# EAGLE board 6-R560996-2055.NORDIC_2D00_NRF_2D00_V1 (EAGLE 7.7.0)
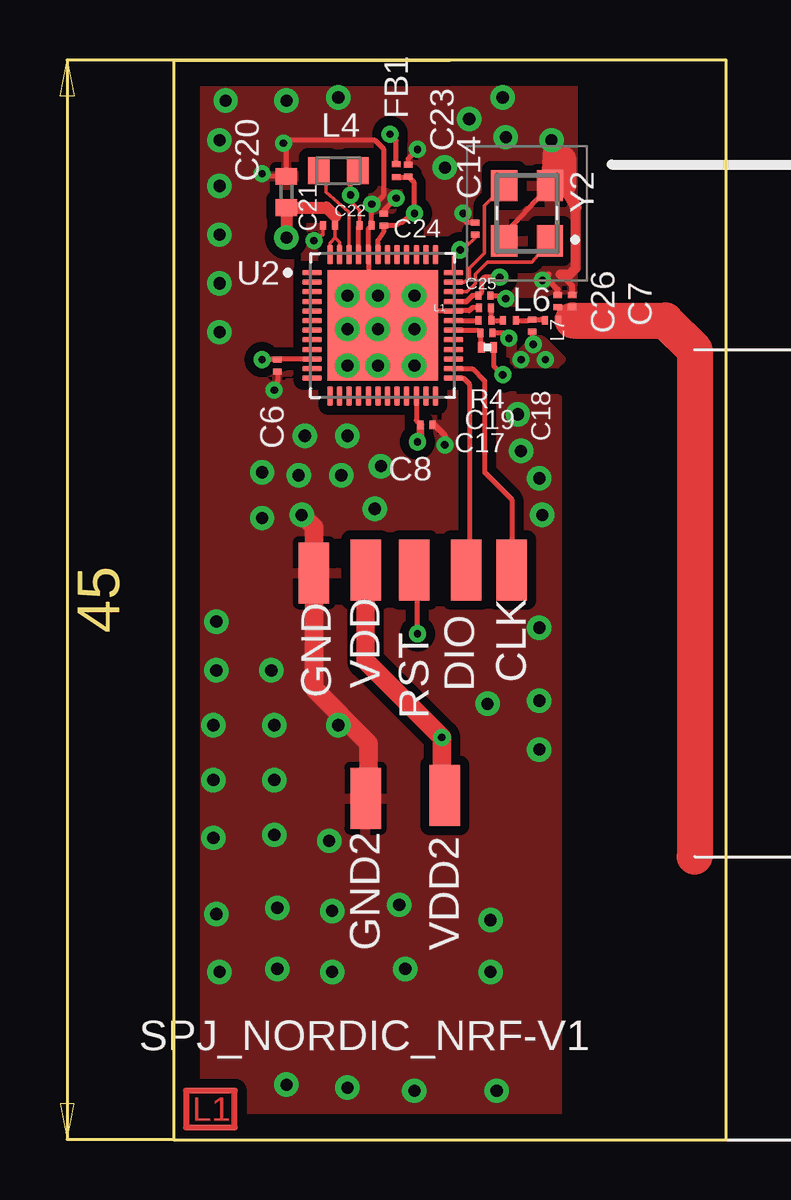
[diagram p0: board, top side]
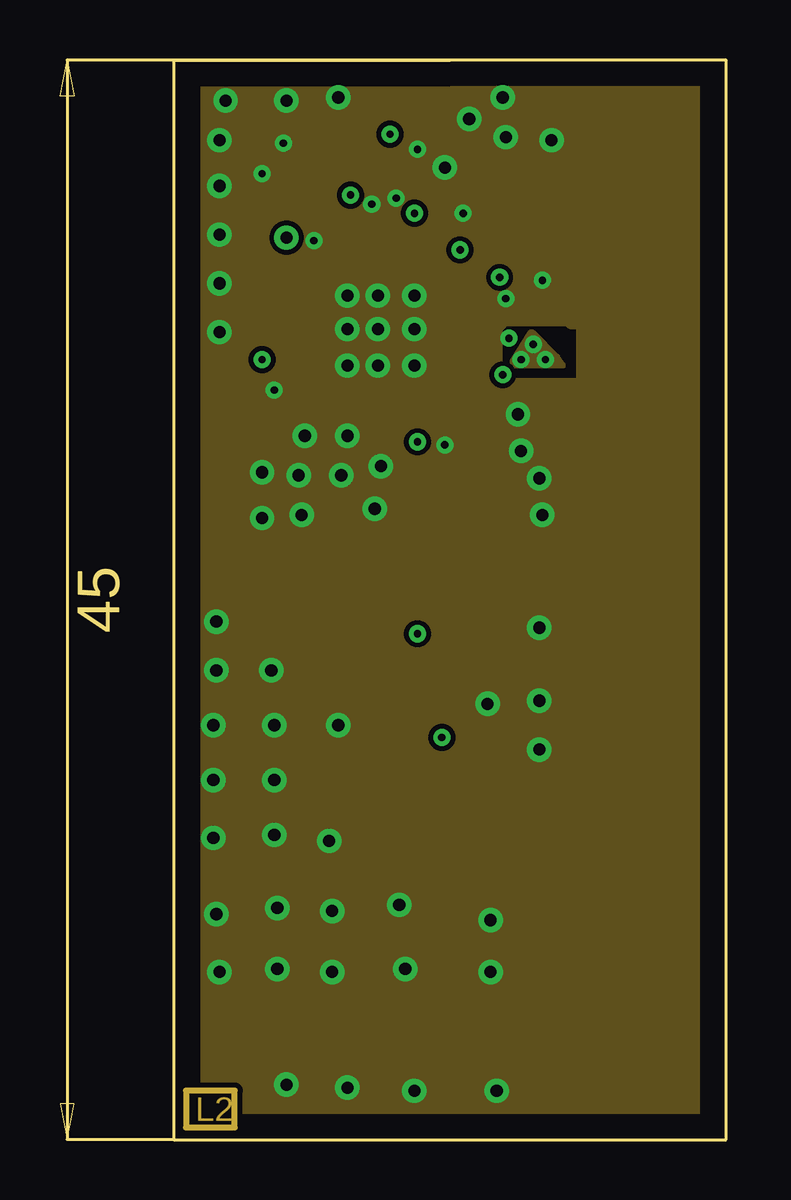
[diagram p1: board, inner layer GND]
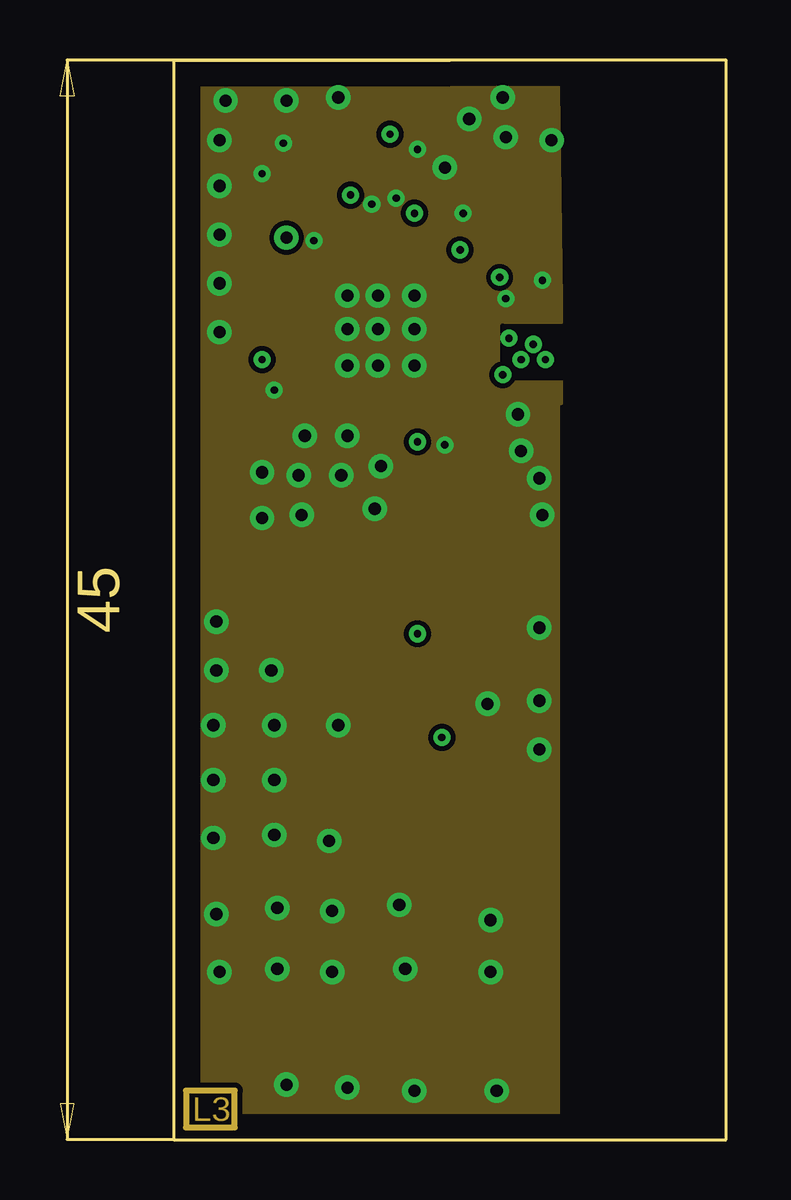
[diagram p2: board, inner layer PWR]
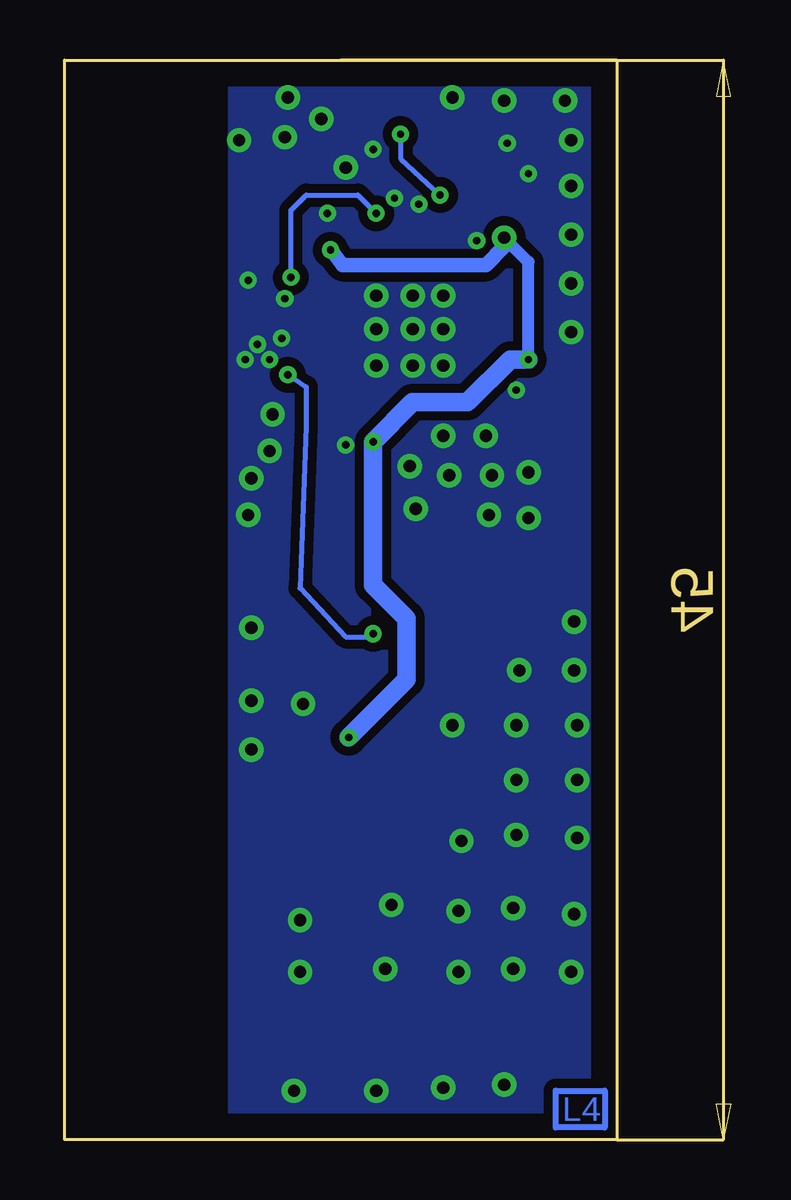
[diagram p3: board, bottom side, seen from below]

Size 27.77 x 45 mm. Coordinates in mm from the lower left corner, seen from the top.
Outline: 27.77,0 27.77,45 4.75,45 4.75,0 27.77,0
Copper layers (1*2+3*16): Top 0.035mm / dielectric 0.5mm / GND 0.035mm / dielectric 0.46mm / PWR 0.035mm / dielectric 0.5mm / Bottom 0.035mm
Design rules "default *": minimum track width 6mil, minimum drill 10mil, track to track 8mil, track to pad 8mil, pad to pad 8mil, via to via 8mil, smd to smd 8mil, copper to edge 40mil, drill to drill 8mil, minimum pad ring 10mil, minimum via ring 8mil, stop-mask expansion 4mil, vias tented up to drill 0mil, thermal gap 10mil

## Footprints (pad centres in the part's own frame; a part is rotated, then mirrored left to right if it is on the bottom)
C0201 = smd 0.25 x 0.35: 1 -0.25,0; 2 0.25,0
C0402 = smd 0.7 x 0.9: 1 -0.65,0; 2 0.65,0
SMD2 = smd 1.27 x 2.54: 1 0,0
L0201 = smd 0.25 x 0.35: 1 -0.275,0; 2 0.275,0
INDC1608X100N = smd 0.89 x 1.11: 1 -0.814,0; 2 0.814,0
R0201 = smd 0.28 x 0.43: 1 -0.255,0; 2 0.255,0
QFN40P600X600X90-49N = smd 0.81 x 0.22: 1 -2.95,2.2; 2 -2.95,1.8; 3 -2.95,1.4; 4 -2.95,1; 5 -2.95,0.6; 6 -2.95,0.2; 7 -2.95,-0.2; 8 -2.95,-0.6; 9 -2.95,-1; 10 -2.95,-1.4; 11 -2.95,-1.8; 12 -2.95,-2.2; 25 2.95,-2.2; 26 2.95,-1.8; 27 2.95,-1.4; 28 2.95,-1; 29 2.95,-0.6; 30 2.95,-0.2; 31 2.95,0.2; 32 2.95,0.6; 33 2.95,1; 34 2.95,1.4; 35 2.95,1.8; 36 2.95,2.2 | smd 0.22 x 0.81: 13 -2.2,-2.95; 14 -1.8,-2.95; 15 -1.4,-2.95; 16 -1,-2.95; 17 -0.6,-2.95; 18 -0.2,-2.95; 19 0.2,-2.95; 20 0.6,-2.95; 21 1,-2.95; 22 1.4,-2.95; 23 1.8,-2.95; 24 2.2,-2.95; 37 2.2,2.95; 38 1.8,2.95; 39 1.4,2.95; 40 1,2.95; 41 0.6,2.95; 42 0.2,2.95; 43 -0.2,2.95; 44 -0.6,2.95; 45 -1,2.95; 46 -1.4,2.95; 47 -1.8,2.95; 48 -2.2,2.95 | smd 4.6 x 4.6: 49 0,0
ABM8AIG12000MHZ12D2ZT = smd 1.3 x 1.1: 1 -1.15,-0.95; 2 1.15,-0.95; 3 1.15,0.95; 4 -1.15,0.95

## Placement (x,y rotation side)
C6  100nF  [C0201]  9.06,32.26 90 top
C7  0.3pF  [C0201]  20.75,34.95 270 top
C8  100nF  [C0201]  15.29,29.79 180 top
C14  100nF  [C0201]  17.32,37.97 270 top
C17  1.5pF  [C0201]  17.72,34.67 0 top
C18  2pF  [C0201]  19.68,33.93 90 top
C19  3.9pF  [C0201]  17.78,33.63 180 top
C20  10uF  [C0402]  9.44,39.5 270 top
C21  100nF  [C0201]  11.22,38.1 0 top
C22  2.2uF  [C0201]  12.75,38.1 180 top
C23  2.2uF  [C0201]  14.52,40.39 270 top
C24  10nF  [C0201]  13.51,38.35 270 top
C25  2.2nF  [C0201]  17.7,35.18 180 top
C26  1.4pF  [C0201]  21.36,34.95 270 top
CLK  [SMD2]  18.84,23.75 0 top
DIO  [SMD2]  16.94,23.75 0 top
FB1  120E/0.2A  [L0201]  14.02,40.39 90 top
GND  [SMD2]  10.59,23.62 0 top
GND2  [SMD2]  12.75,14.22 0 top
L1  2.7nH  [L0201]  17.72,34.14 0 top
L4  4.7uH  [INDC1608X100N]  11.6,40.39 180 top
L6  3.5nH  [L0201]  18.74,34.14 0 top
L7  3.5nH  [L0201]  20.49,34.14 0 top
R4  1K  [R0201]  17.83,33.02 180 top
RST  [SMD2]  14.78,23.75 0 top
U2  NRF54L15-QFAA-R  [QFN40P600X600X90-49N]  13.46,33.93 0 top
VDD  [SMD2]  12.75,23.75 0 top
VDD2  [SMD2]  16.05,14.35 0 top
Y2  ABM8AIG-32.000MHZ-1Z-T  [ABM8AIG12000MHZ12D2ZT]  19.48,38.61 90 top

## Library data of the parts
C6-C8 C14 C17-C26 FB1 L1 L4 L6 L7 R4 = rcl
CLK DIO GND GND2 RST VDD VDD2 = wirepad
U2 = NRF54L15-QFAA-R; MANUFACTURER: Nordic; MAXIMUM_PACKAGE_HEIGHT: 0.9mm; PARTREV: 0.8; STANDARD: IPC-7351B
Y2 = ABM8AIG-32.000MHZ-1Z-T; DESCRIPTION: Crystals 18pF 32MHz 10ppm AEC-Q200 -40C +125C; HEIGHT: 0.8mm; MANUFACTURER_NAME: ABRACON; MANUFACTURER_PART_NUMBER: ABM8AIG-32.000MHZ-1Z-T; MOUSER_PART_NUMBER: 815-M8AIG-32-1ZT; MOUSER_PRICE-STOCK: https://www.mouser.com/Search/Refine.aspx?Keyword=815-M8AIG-32-1ZT

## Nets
GND: C6.1 C7.1 C8.1 C14.1 C17.1 C18.1 C19.1 C20.1 C21.1 C22.1 C23.1 C24.1 C25.1 C26.1 GND2.1 GND.1 U2.32 U2.44 U2.49 Y2.2 Y2.4
N$3: L1.1 U2.31
N$12: U2.34 Y2.1
N$14: U2.35 Y2.3
N$16: C19.2 R4.2 U2.30
N$18: L4.2 U2.46
N$19: C22.2 FB1.2 L4.1 U2.45
N$20: C18.2 L6.2 L7.1
N$21: C23.2 C24.2 C25.2 FB1.1 U2.33 U2.43
N$22: C17.2 L1.2 L6.1
P2.00: U2.11
RF: C7.2 C26.2 L7.2
RST: R4.1 RST.1
SWDCLK: CLK.1 U2.26
SWDIO: DIO.1 U2.25
VDD: C6.2 C8.2 C14.2 C20.2 C21.2 U2.10 U2.22 U2.36 U2.47 U2.48 VDD2.1 VDD.1

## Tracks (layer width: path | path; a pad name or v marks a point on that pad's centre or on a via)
GND  (via drill 0.3 pad 0.61, 0.51 pad 1.02)
  Top 0.152: C21.1 10.97,37.72 10.59,37.59 v10.59,37.47
  Top 0.203: C17.1 17.19,34.67 17.06,34.54 16.42,34.54 U2.32 14.06,34.53 U2.49 12.86,34.53 U2.44 12.86,37.96 C22.1 v13,38.98 v13,38.99 13.13,38.99 13.51,39.37 13.51,41.27 13.13,41.66 9.44,41.66 v9.32,41.53 9.44,41.4 C20.1 8.54,40.15 v8.43,40.26 | Y2.4 18.65,37.86 Y2.2 | C14.1 16.94,38.22 16.81,38.35 v16.81,38.61 | C25.1 18.46,35.18 v18.59,35.05 | C19.1 18.49,33.63 v18.71,33.4 | C18.1 19.68,33.2 v19.73,33.15 19.73,33.02 | C24.1 13.51,38.73 v14.02,39.24 | C23.1 14.52,40.89 v14.91,41.27 | C6.1 9.06,31.62 v8.94,31.24
  Top 0.254: C7.1 20.75,35.43 20.37,35.81 v20.11,35.81 20.37,36.07 | C26.1 21.36,35.59 20.87,36.07 | C8.1 15.59,29.79 16.05,29.34 v16.05,28.96
  Top 0.406: 20.87,36.07 21.26,36.07 21.51,36.32 21.51,38.86 | 21,40.89 v20.49,41.66
  Top 0.508: 21.51,38.86 21,39.75
  Top 0.762: Y2.2 20.55,41.59 v20.49,41.66 | GND2.1 12.87,14.35 12.87,16.51 10.59,18.8 GND.1 10.59,25.53 v10.08,26.04
  Top 1.016: 21,39.75 21,40.89
  other vias: 19.22,32.51 20.24,32.51 18.46,43.43 18.59,41.78 17.06,42.55 16.05,40.51 11.6,43.43 9.44,43.31 6.9,43.31 6.65,41.66 6.65,39.75 6.65,37.72 6.65,35.69 6.65,33.66 10.21,29.34 11.98,29.34 13.38,28.07 13.13,26.29 11.73,27.69 9.95,27.69 6.52,21.59 6.52,19.56 8.81,19.56 6.4,17.27 8.94,17.27 11.6,17.27 6.4,14.99 8.94,14.99 6.4,12.57 8.94,12.7 11.98,35.18 13.25,35.18 14.78,35.18 14.78,33.78 13.25,33.78 11.98,33.78 11.98,32.26 13.25,32.26 14.78,32.26 19.1,30.23 19.22,28.7 19.98,27.56 20.11,26.04 19.98,21.34 17.83,18.16 19.98,18.29 19.98,16.26 6.52,9.4 9.06,9.65 6.65,6.99 9.06,7.11 11.35,6.99 11.35,9.53 11.22,12.45 14.14,9.78 14.4,7.11 17.95,9.14 17.95,6.99 18.21,2.03 14.78,2.03 11.98,2.16 9.44,2.29 8.43,25.91 8.43,27.81
  pour Top (isolate 0.381): 20.11,44.58 5.38,44.45 5.38,0.38 20.75,0.38 20.75,30.86 18.84,30.86 18.84,35.31 21.38,35.31 21.38,44.32
  pour Bottom (isolate 0.381): 20.75,44.07 5.76,43.94 5.76,0.89 20.75,0.89
  pour GND: 27.73,44.07 5.51,43.94 5.51,0.89 27.61,0.89 27.61,31.62 18.46,31.62 18.33,31.75 18.33,33.78 18.59,34.04 21.13,34.04 21.26,33.91 21.64,33.91 21.64,31.75 27.1,31.75 27.35,32.13
  pour PWR: 20.75,43.81 5.89,43.81 5.89,1.14 20.75,1.14 20.75,30.73 20.87,30.73 20.87,34.92
  pour Top (no thermals): 19.6,33.27 18.84,32.51 18.84,32.38 18.97,32.26 20.75,32.26 21,32.51 20.11,33.4 19.73,33.4
  pour GND (no thermals): 19.73,33.66 19.6,33.66 18.71,32.26 21,32.26 20.75,32.64
N$1
  Top 0.254: 7.29,2.03 5.25,2.03 5.25,0.51 7.29,0.51 7.29,2.03
N$2
  GND 0.254: 7.29,2.03 5.25,2.03 5.25,0.51 7.29,0.51 7.29,2.03
N$3
  Top 0.203: U2.31 L1.1
N$4
  PWR 0.254: 7.29,2.03 5.25,2.03 5.25,0.51 7.29,0.51 7.29,2.03
N$5
  Bottom 0.254: 7.29,2.03 5.25,2.03 5.25,0.51 7.29,0.51 7.29,2.03
N$6
  cutout PWR: 18.46,33.91 21,33.91 21,31.75 18.46,31.75
N$12
  Top 0.152: U2.34 16.96,35.33 17.32,35.69 17.32,36.07 17.83,36.58 19.67,36.58 Y2.1
N$14
  Top 0.152: U2.35 16.86,35.73 17.06,35.94 17.06,36.32 17.7,36.96 17.7,38.93 Y2.3
N$16
  Top 0.203: U2.30 17.42,33.73 C19.2 17.52,33.07 R4.2
N$18
  Top 0.152: U2.46 12.06,38.66 11.09,39.5 11.09,40.21 L4.2
N$19  (via drill 0.3 pad 0.61)
  Top 0.152: C22.2 12.5,38.73 12.11,39.12 v12.12,39.37
  Top 0.203: U2.45 12.46,38.06 C22.2 | FB1.2 14.02,41.66 v13.76,41.91 | v12.12,39.37 12.12,40.01 12.37,40.26 12.5,40.34 L4.1
  Bottom 0.203: v13.76,41.91 13.76,40.89 v12.12,39.37
N$20
  Top 0.203: L6.2 19.51,34.14 C18.2 20.04,34.18 L7.1
N$21  (via drill 0.3 pad 0.61)
  Top 0.203: 16.95,34.93 16.94,34.92 16.42,34.92 U2.33 16.95,34.93 | 16.95,34.93 17.19,35.18 C25.2 17.57,35.3 17.57,35.81 17.7,35.94 v18.33,35.94 | v14.78,38.61 14.02,38.1 C24.2 13.51,37.85 13.26,37.47 U2.43 | 14.27,38.23 v14.78,38.61 | v14.78,38.61 14.78,39.88 C23.2 14.5,40.11 FB1.1
  Bottom 0.203: v18.33,35.94 18.33,38.73 17.7,39.37 15.54,39.37 v14.78,38.61
N$22
  Top 0.203: C17.2 18,34.65 L1.2 L6.1
RF
  Top 0.203: L7.2 20.77,34.37 C26.2 C7.2
  Top 0.254: 21.38,34.14 21.31,34.14 C7.2
  Top 1.5: 21.38,34.14 25.24,34.14 26.46,32.92 26.46,11.79
RST  (via drill 0.3 pad 0.61)
  Top 0.203: R4.1 18.08,32.26 v18.46,31.88 | v14.91,21.08 14.91,23.62 RST.1
  Bottom 0.203: v18.46,31.88 17.7,31.37 17.7,29.72 17.95,22.99 16.05,20.95 15.03,20.95 v14.91,21.08
SWDCLK
  Top 0.203: U2.26 17.19,32.13 17.7,31.62 17.7,27.81 18.84,26.67 CLK.1
SWDIO
  Top 0.203: U2.25 16.83,31.73 17.06,31.5 17.06,23.88 DIO.1
VDD  (via drill 0.3 pad 0.61, 0.51 pad 1.02)
  Top 0.152: C14.2 17.32,37.59 16.94,37.21 16.81,37.21 v16.68,37.08 16.41,36.81 U2.36 | U2.48 11.26,37.37 11.48,37.59 | 11.48,37.59 C21.2 | U2.47 11.66,37.41 11.48,37.59
  Top 0.203: U2.22 14.86,29.97 C8.2 | C6.2 v8.43,32.51 8.45,32.53 U2.10
  Top 0.254: 11.48,38.48 C21.2
  Top 0.305: C8.2 15.04,29.21 v14.91,29.08
  Top 0.508: 11.48,38.48 11.11,38.85 C20.2 v9.44,37.59
  Top 0.762: VDD2.1 15.92,14.48 v15.92,16.76 12.75,19.94 VDD.1
  Bottom 0.508: v8.43,32.51 8.43,36.58 v9.44,37.59
  Bottom 0.61: v16.68,37.08 16.56,36.96 16.18,36.45 10.21,36.45 9.44,37.21 v9.44,37.59
  Bottom 0.762: v15.92,16.76 13.51,19.18 13.51,21.72 14.91,23.11 v14.91,29.08 13.25,30.73 10.97,30.73 9.19,32.51 v8.43,32.51

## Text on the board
Top: L1
GND: L2
PWR: L3
Bottom: L4
tNames: SPJ_NORDIC_NRF-V1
